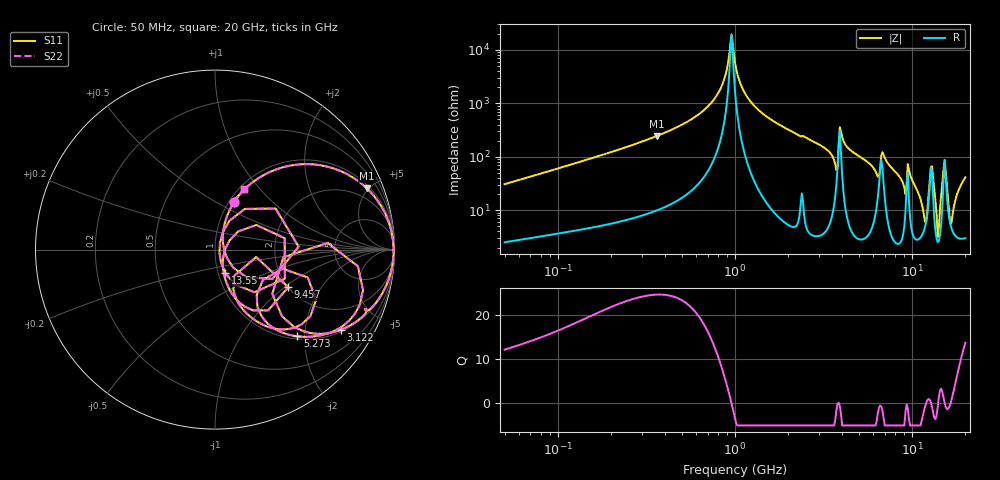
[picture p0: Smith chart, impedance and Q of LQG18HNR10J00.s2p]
!Murata Part Number: LQG18HNR10J00
!These Parameters are Measured in Series Mode Connection
!  o--[Z]--o
!Port1  Port2
!  o-------o
!Freq. Start=50[MHz] Stop=20[GHz], 401[Steps]
# Hz S RI R 50
!Freq.(Hz) S11(Real) S11(Imag) S21(Real) S21(Imag) S12(Real) S12(Imag) S22(Real) S22(Imag)
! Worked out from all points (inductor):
!   401 points, 50 MHz to 20 GHz, reference 50 ohm
!   read as one part in series: L = 96.3 nH near 51.52 MHz
!   highest Q = 24.7 at 361.1 MHz (marker M1), where L = 108 nH
!   self-resonance near 956.1 MHz
!   S11 on the Smith chart (normalised r, x): 50 MHz: 1.05, +0.61; 3.122 GHz: 1.07, -3.10; 5.273 GHz: 1.06, -1.84; 9.457 GHz: 2.00, -1.06; 13.55 GHz: 1.08, -0.29; 20 GHz: 1.06, +0.82
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5e7  0.1044 0.2674  0.8956 -0.2674  0.8956 -0.2674  0.1044 0.2674
1.364002e8  0.4094 0.466  0.5906 -0.466  0.5906 -0.466  0.4094 0.466
3.611186e8  0.8467 0.3405  0.1533 -0.3405  0.1533 -0.3405  0.8467 0.3405
3.721004e8  0.8562 0.3312  0.1438 -0.3312  0.1438 -0.3312  0.8562 0.3312
6.980337e8  0.9798 0.1135  0.0202 -0.1135  0.0202 -0.1135  0.9798 0.1135
8.480927e8  0.9924 0.0434  0.0076 -0.0434  0.0076 -0.0434  0.9924 0.0434
9.418449e8  0.9948 0.00548  0.00521 -0.00548  0.00521 -0.00548  0.9948 0.00548
1e9  0.9948 -0.0163  0.0052 0.0163  0.0052 0.0163  0.9948 -0.0163
1.309461e9  0.982 -0.1161  0.018 0.1161  0.018 0.1161  0.982 -0.1161
2.728004e9  0.793 -0.3967  0.207 0.3967  0.207 0.3967  0.793 -0.3967
3.121702e9  0.7018 -0.4463  0.2982 0.4463  0.2982 0.4463  0.7018 -0.4463
3.850025e9  0.6282 0.0367  0.3718 -0.0367  0.3718 -0.0367  0.6282 0.0367
5.273168e9  0.4595 -0.4831  0.5405 0.4831  0.5405 0.4831  0.4595 -0.4831
7.442007e9  0.3347 -0.441  0.6653 0.441  0.6653 0.441  0.3347 -0.441
9.457416e9  0.4079 -0.2097  0.5921 0.2097  0.5921 0.2097  0.4079 -0.2097
1.183995e10  0.0479 -0.0319  0.9521 0.0319  0.9521 0.0319  0.0479 -0.0319
1.295331e10  0.3889 -0.1621  0.6111 0.1621  0.6111 0.1621  0.3889 -0.1621
1.354865e10  0.0577 -0.1315  0.9423 0.1315  0.9423 0.1315  0.0577 -0.1315
1.417136e10  0.0275 0.0367  0.9725 -0.0367  0.9725 -0.0367  0.0275 0.0367
1.527346e10  0.4658 0.0164  0.5342 -0.0164  0.5342 -0.0164  0.4658 0.0164
1.670968e10  0.0447 0.0354  0.9553 -0.0354  0.9553 -0.0354  0.0447 0.0354
2e10  0.1632 0.335  0.8368 -0.335  0.8368 -0.335  0.1632 0.335
